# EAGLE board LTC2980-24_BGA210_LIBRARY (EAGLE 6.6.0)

No outline drawn. Coordinates in mm, seen from the top.
Copper layers (1*2+15*16): Top 0.06mm / dielectric 0.2mm / Route2 0.035mm / dielectric 0.15mm / Route15 0.035mm / dielectric 0.2mm / Bottom 0.06mm
Design rules "default": minimum track width 10mil, minimum drill 24mil, track to track 8mil, track to pad 8mil, pad to pad 8mil, via to via 8mil, smd to smd 8mil, copper to edge 40mil, drill to drill 8mil, minimum pad ring 10mil, minimum via ring 8mil, stop-mask expansion 4mil, vias tented up to drill 0mil, thermal gap 10mil

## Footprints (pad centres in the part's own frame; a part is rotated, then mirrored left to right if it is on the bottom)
BGA210 = smd 0.4 x 0.4: A1 -8,-3.6; A2 -8,-2.8; A3 -8,-2; A4 -8,-1.2; A5 -8,-0.4; A6 -8,0.4; A7 -8,1.2; A8 -8,2; A9 -8,2.8; A10 -8,3.6; B1 -7.2,-3.6; B2 -7.2,-2.8; B3 -7.2,-2; B4 -7.2,-1.2; B5 -7.2,-0.4; B6 -7.2,0.4; B7 -7.2,1.2; B8 -7.2,2; B9 -7.2,2.8; B10 -7.2,3.6; C1 -6.4,-3.6; C2 -6.4,-2.8; C3 -6.4,-2; C4 -6.4,-1.2; C5 -6.4,-0.4; C6 -6.4,0.4; C7 -6.4,1.2; C8 -6.4,2; C9 -6.4,2.8; C10 -6.4,3.6; D1 -5.6,-3.6; D2 -5.6,-2.8; D3 -5.6,-2; D4 -5.6,-1.2; D5 -5.6,-0.4; D6 -5.6,0.4; D7 -5.6,1.2; D8 -5.6,2; D9 -5.6,2.8; D10 -5.6,3.6; E1 -4.8,-3.6; E2 -4.8,-2.8; E3 -4.8,-2; E4 -4.8,-1.2; E5 -4.8,-0.4; E6 -4.8,0.4; E7 -4.8,1.2; E8 -4.8,2; E9 -4.8,2.8; E10 -4.8,3.6; F1 -4,-3.6; F2 -4,-2.8; F3 -4,-2; F4 -4,-1.2; F5 -4,-0.4; F6 -4,0.4; F7 -4,1.2; F8 -4,2; F9 -4,2.8; F10 -4,3.6; G1 -3.2,-3.6; G2 -3.2,-2.8; G3 -3.2,-2; G4 -3.2,-1.2; G5 -3.2,-0.4; G6 -3.2,0.4; G7 -3.2,1.2; G8 -3.2,2; G9 -3.2,2.8; G10 -3.2,3.6; H1 -2.4,-3.6; H2 -2.4,-2.8; H3 -2.4,-2; H4 -2.4,-1.2; H5 -2.4,-0.4; H6 -2.4,0.4; H7 -2.4,1.2; H8 -2.4,2; H9 -2.4,2.8; H10 -2.4,3.6; J1 -1.6,-3.6; J2 -1.6,-2.8; J3 -1.6,-2; J4 -1.6,-1.2; J5 -1.6,-0.4; J6 -1.6,0.4; J7 -1.6,1.2; J8 -1.6,2; J9 -1.6,2.8; J10 -1.6,3.6; K1 -0.8,-3.6; K2 -0.8,-2.8; K3 -0.8,-2; K4 -0.8,-1.2; K5 -0.8,-0.4; K6 -0.8,0.4; K7 -0.8,1.2; K8 -0.8,2; K9 -0.8,2.8; K10 -0.8,3.6; L1 0,-3.6; L2 0,-2.8; L3 0,-2; L4 0,-1.2; L5 0,-0.4; L6 0,0.4; L7 0,1.2; L8 0,2; L9 0,2.8; L10 0,3.6; M1 0.8,-3.6; M2 0.8,-2.8; M3 0.8,-2; M4 0.8,-1.2; M5 0.8,-0.4; M6 0.8,0.4; M7 0.8,1.2; M8 0.8,2; M9 0.8,2.8; M10 0.8,3.6; N1 1.6,-3.6; N2 1.6,-2.8; N3 1.6,-2; N4 1.6,-1.2; N5 1.6,-0.4; N6 1.6,0.4; N7 1.6,1.2; N8 1.6,2; N9 1.6,2.8; N10 1.6,3.6; P1 2.4,-3.6; P2 2.4,-2.8; P3 2.4,-2; P4 2.4,-1.2; P5 2.4,-0.4; P6 2.4,0.4; P7 2.4,1.2; P8 2.4,2; P9 2.4,2.8; P10 2.4,3.6; R1 3.2,-3.6; R2 3.2,-2.8; R3 3.2,-2; R4 3.2,-1.2; R5 3.2,-0.4; R6 3.2,0.4; R7 3.2,1.2; R8 3.2,2; R9 3.2,2.8; R10 3.2,3.6; T1 4,-3.6; T2 4,-2.8; T3 4,-2; T4 4,-1.2; T5 4,-0.4; T6 4,0.4; T7 4,1.2; T8 4,2; T9 4,2.8; T10 4,3.6; U1 4.8,-3.6; U2 4.8,-2.8; U3 4.8,-2; U4 4.8,-1.2; U5 4.8,-0.4; U6 4.8,0.4; U7 4.8,1.2; U8 4.8,2; U9 4.8,2.8; U10 4.8,3.6; W1 5.6,-3.6; W2 5.6,-2.8; W3 5.6,-2; W4 5.6,-1.2; W5 5.6,-0.4; W6 5.6,0.4; W7 5.6,1.2; W8 5.6,2; W9 5.6,2.8; W10 5.6,3.6; X1 6.4,-3.6; X2 6.4,-2.8; X3 6.4,-2; X4 6.4,-1.2; X5 6.4,-0.4; X6 6.4,0.4; X7 6.4,1.2; X8 6.4,2; X9 6.4,2.8; X10 6.4,3.6; Y1 7.2,-3.6; Y2 7.2,-2.8; Y3 7.2,-2; Y4 7.2,-1.2; Y5 7.2,-0.4; Y6 7.2,0.4; Y7 7.2,1.2; Y8 7.2,2; Y9 7.2,2.8; Y10 7.2,3.6; Z1 8,-3.6; Z2 8,-2.8; Z3 8,-2; Z4 8,-1.2; Z5 8,-0.4; Z6 8,0.4; Z7 8,1.2; Z8 8,2; Z9 8,2.8; Z10 8,3.6

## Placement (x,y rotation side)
E$1  [BGA210]  8,3.6 0 top

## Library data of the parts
E$1 = linear-technology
